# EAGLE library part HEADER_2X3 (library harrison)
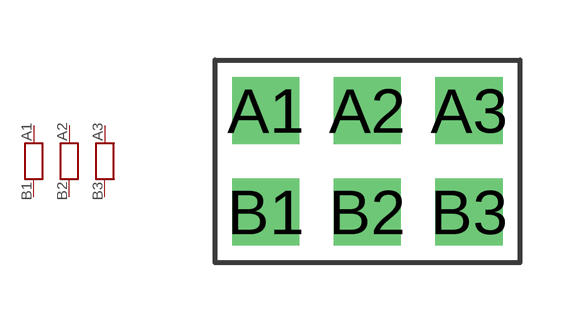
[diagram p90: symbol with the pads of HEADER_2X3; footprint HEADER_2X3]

Designator prefix S

## HEADER_2X3  [HEADER_2X3]
A1  A1  pas
A2  A2  pas
A3  A3  pas
B1  B1  pas
B2  B2  pas
B3  B3  pas

## Footprint HEADER_2X3 (pad centres in mm)
drill 0.813 pad 1.676 square: A1 -2.54,1.27; A2 0,1.27; A3 2.54,1.27; B1 -2.54,-1.27; B2 0,-1.27; B3 2.54,-1.27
